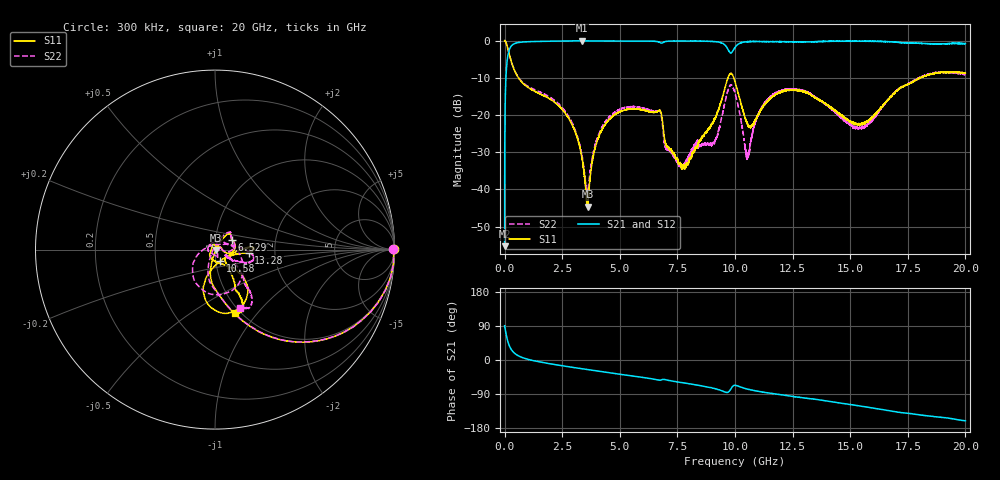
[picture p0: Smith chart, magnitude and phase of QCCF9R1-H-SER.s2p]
!QCCF9R1
!Johanson Technology Inc.
!www.johansontechnology.com
!Test Board Conditions:
!Substrate Type  RO4350B
!Substrate Thickness  10 mil
!Substrate Dk  3.66
!TL Type: GCPW
!TL Trace Width  21 mil
!TL Gap  20 mil
!Electrode orientation  Horizontal
!DUT TOPOLOGY	SERIES
!Mounting Pad LxW  16x21 mil
# MHz S  dB  R 50
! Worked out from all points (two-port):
!   20001 points, 300 kHz to 20 GHz, reference 50 ohm
!   highest |S21| = -0.06 dB at 3.37 GHz (marker M1); lowest = -55.2 dB at 300 kHz (marker M2)
!   |S21| within 3 dB of the highest: 174.3 MHz to 9.761 GHz (9.587 GHz wide, 193 % of centre); 9.88 GHz to end of sweep
!   lowest |S11| = -44.6 dB at 3.599 GHz (marker M3), VSWR 1.01, Z = 50.6 - j0.172 ohm
!   |S11| at or under -10 dB: 598.3 MHz to 9.698 GHz (9.1 GHz wide, 177 % of centre); 9.943 GHz to 18.06 GHz (8.115 GHz wide, 58 % of centre); 18.05984 GHz to 18.06009 GHz (251.3 kHz wide, 0.00139 % of centre)
!   |S22| runs from -41.2 to 0.0 dB; largest |S21 - S12| = 0.03
!   S11 on the Smith chart (normalised r, x): 300 kHz: open; 6.529 GHz: 1.20, +0.14; 10.58 GHz: 1.05, -0.14; 13.28 GHz: 1.46, -0.06; 20 GHz: 0.94, -0.76
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0.3  -0.04 0.1  -55.24 90.4  -55.36 89.5  -0.06 0.1
108.298  -1.43 -33.4  -5.51 56.2  -5.53 56.4  -1.45 -33.4
274.296  -5.30 -60.0  -1.59 29.3  -1.58 29.4  -5.30 -59.8
2603.261  -19.28 -103.0  -0.13 -16.1  -0.13 -16.1  -18.80 -109.7
3334.25  -30.66 -100.5  -0.07 -23.0  -0.07 -23.0  -30.18 -130.6
3370.249  -31.79 -99.0  -0.06 -23.3  -0.07 -23.3  -31.29 -132.6
3599.246  -44.61 -16.9  -0.08 -25.4  -0.08 -25.4  -40.67 144.4
4460.233  -21.79 54.1  -0.11 -33.1  -0.10 -33.1  -21.11 60.2
6529.202  -19.25 30.8  -0.22 -51.2  -0.23 -51.2  -19.00 36.0
6667.2  -18.93 22.4  -0.35 -52.9  -0.36 -52.8  -18.87 27.3
7019.195  -28.32 3.3  -0.24 -52.5  -0.25 -52.6  -28.98 15.5
7773.183  -33.55 69.2  -0.15 -60.3  -0.15 -60.4  -33.49 -31.6
9134.163  -20.96 -63.6  -0.29 -75.7  -0.29 -75.6  -27.05 78.7
9632.156  -11.22 -48.8  -1.73 -85.5  -1.73 -85.1  -14.76 -29.4
10000.15  -11.01 -101.3  -1.86 -66.9  -1.84 -66.8  -14.12 -127.6
10584.14  -22.95 -66.7  -0.31 -77.6  -0.29 -77.2  -30.67 78.4
11478.13  -15.86 1.2  -0.32 -87.1  -0.26 -87.4  -15.47 -0.5
13278.1  -14.48 -5.6  -0.34 -102.3  -0.34 -102.5  -14.39 -23.7
13334.1  -14.82 -6.0  -0.36 -102.6  -0.40 -102.7  -14.54 -23.0
15408.07  -22.45 -39.2  -0.17 -121.3  -0.19 -121.0  -23.46 -28.7
16667.05  -15.85 -56.6  -0.32 -133.5  -0.28 -134.1  -15.61 -38.0
20000  -8.72 -72.9  -0.85 -160.6  -0.69 -159.3  -9.09 -67.1
